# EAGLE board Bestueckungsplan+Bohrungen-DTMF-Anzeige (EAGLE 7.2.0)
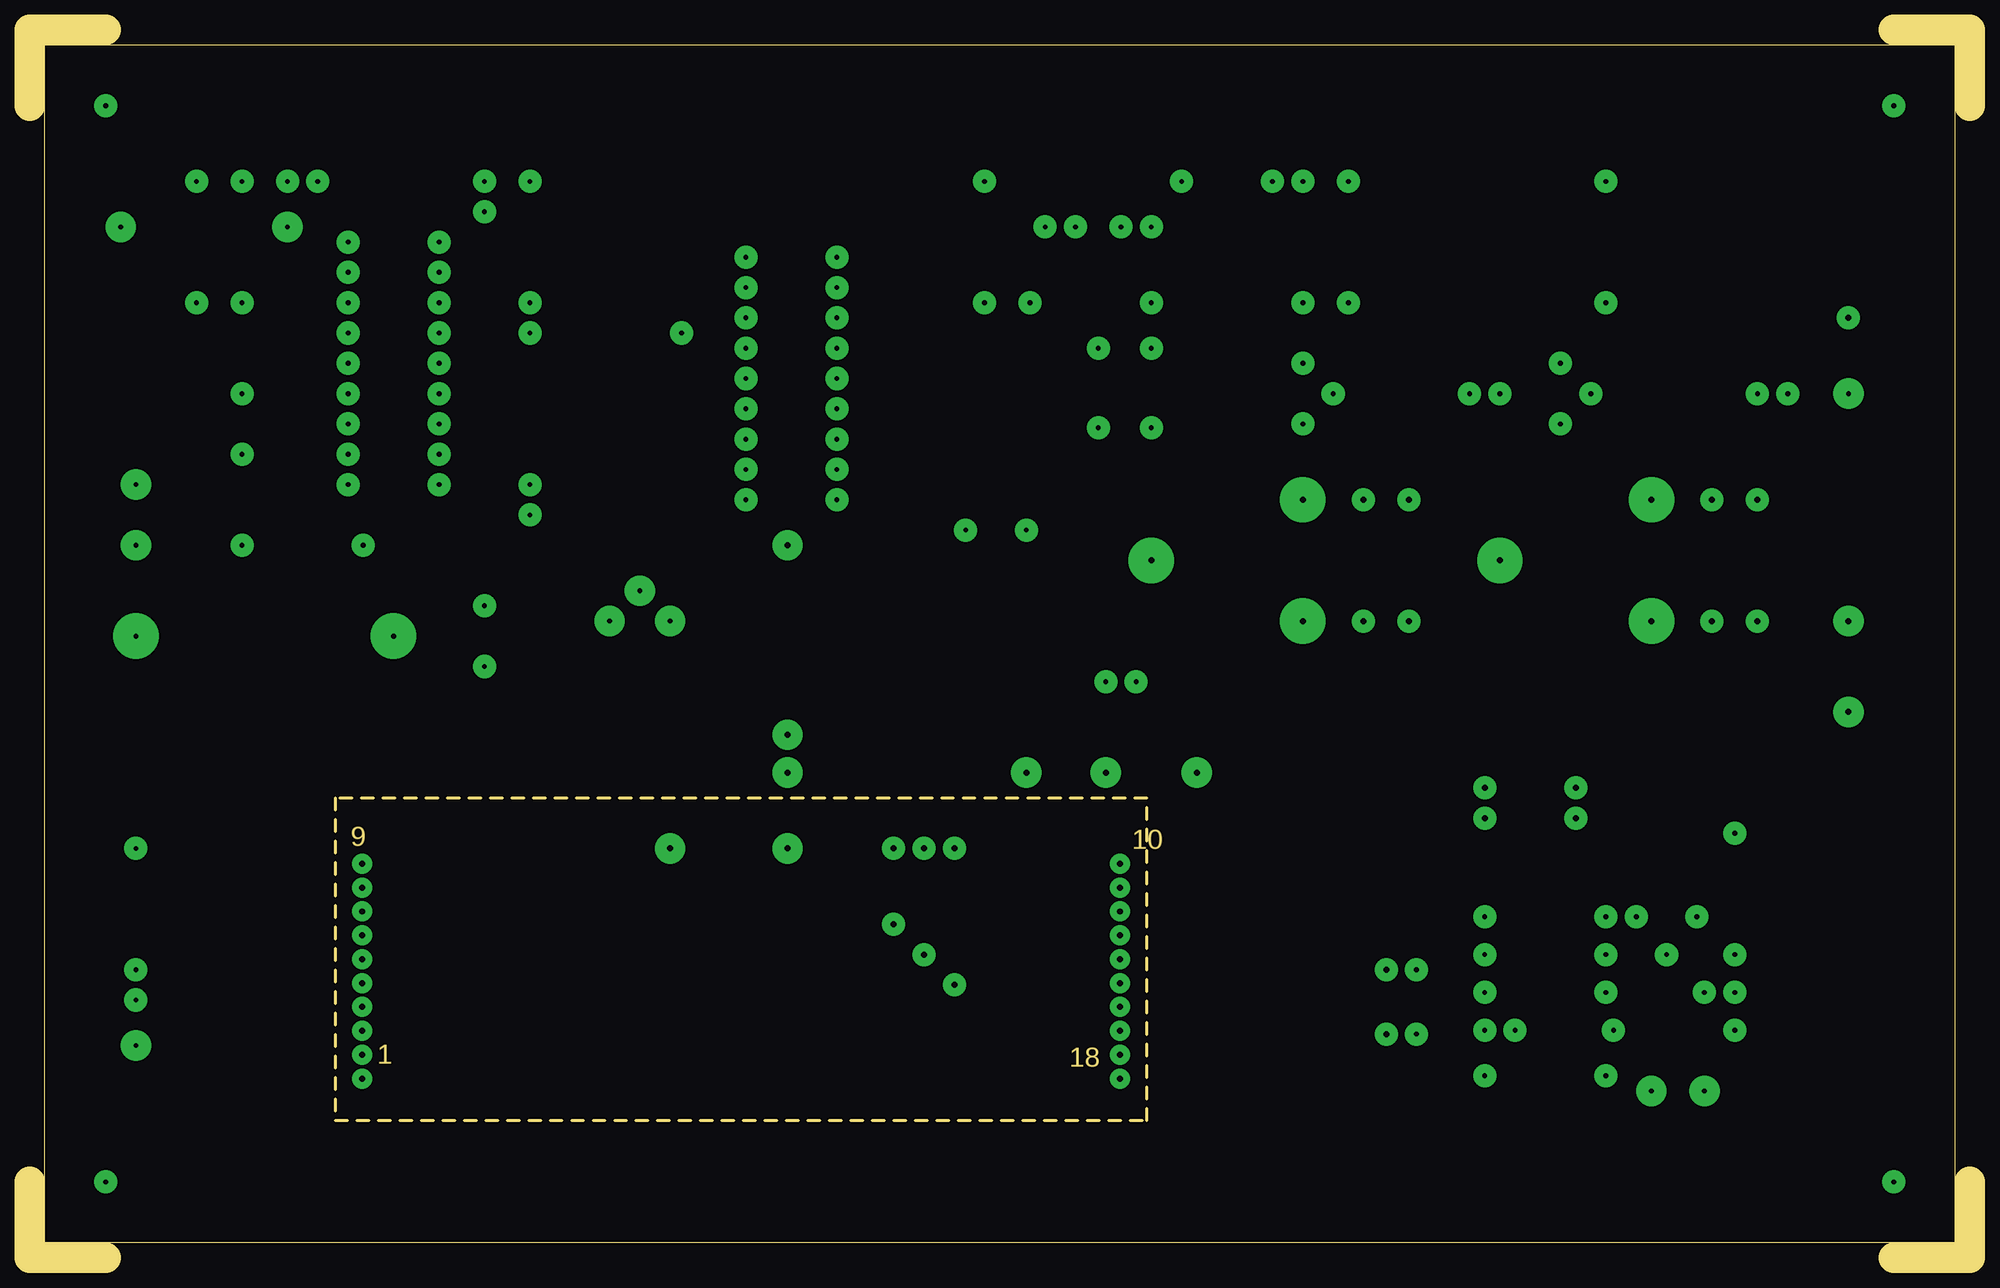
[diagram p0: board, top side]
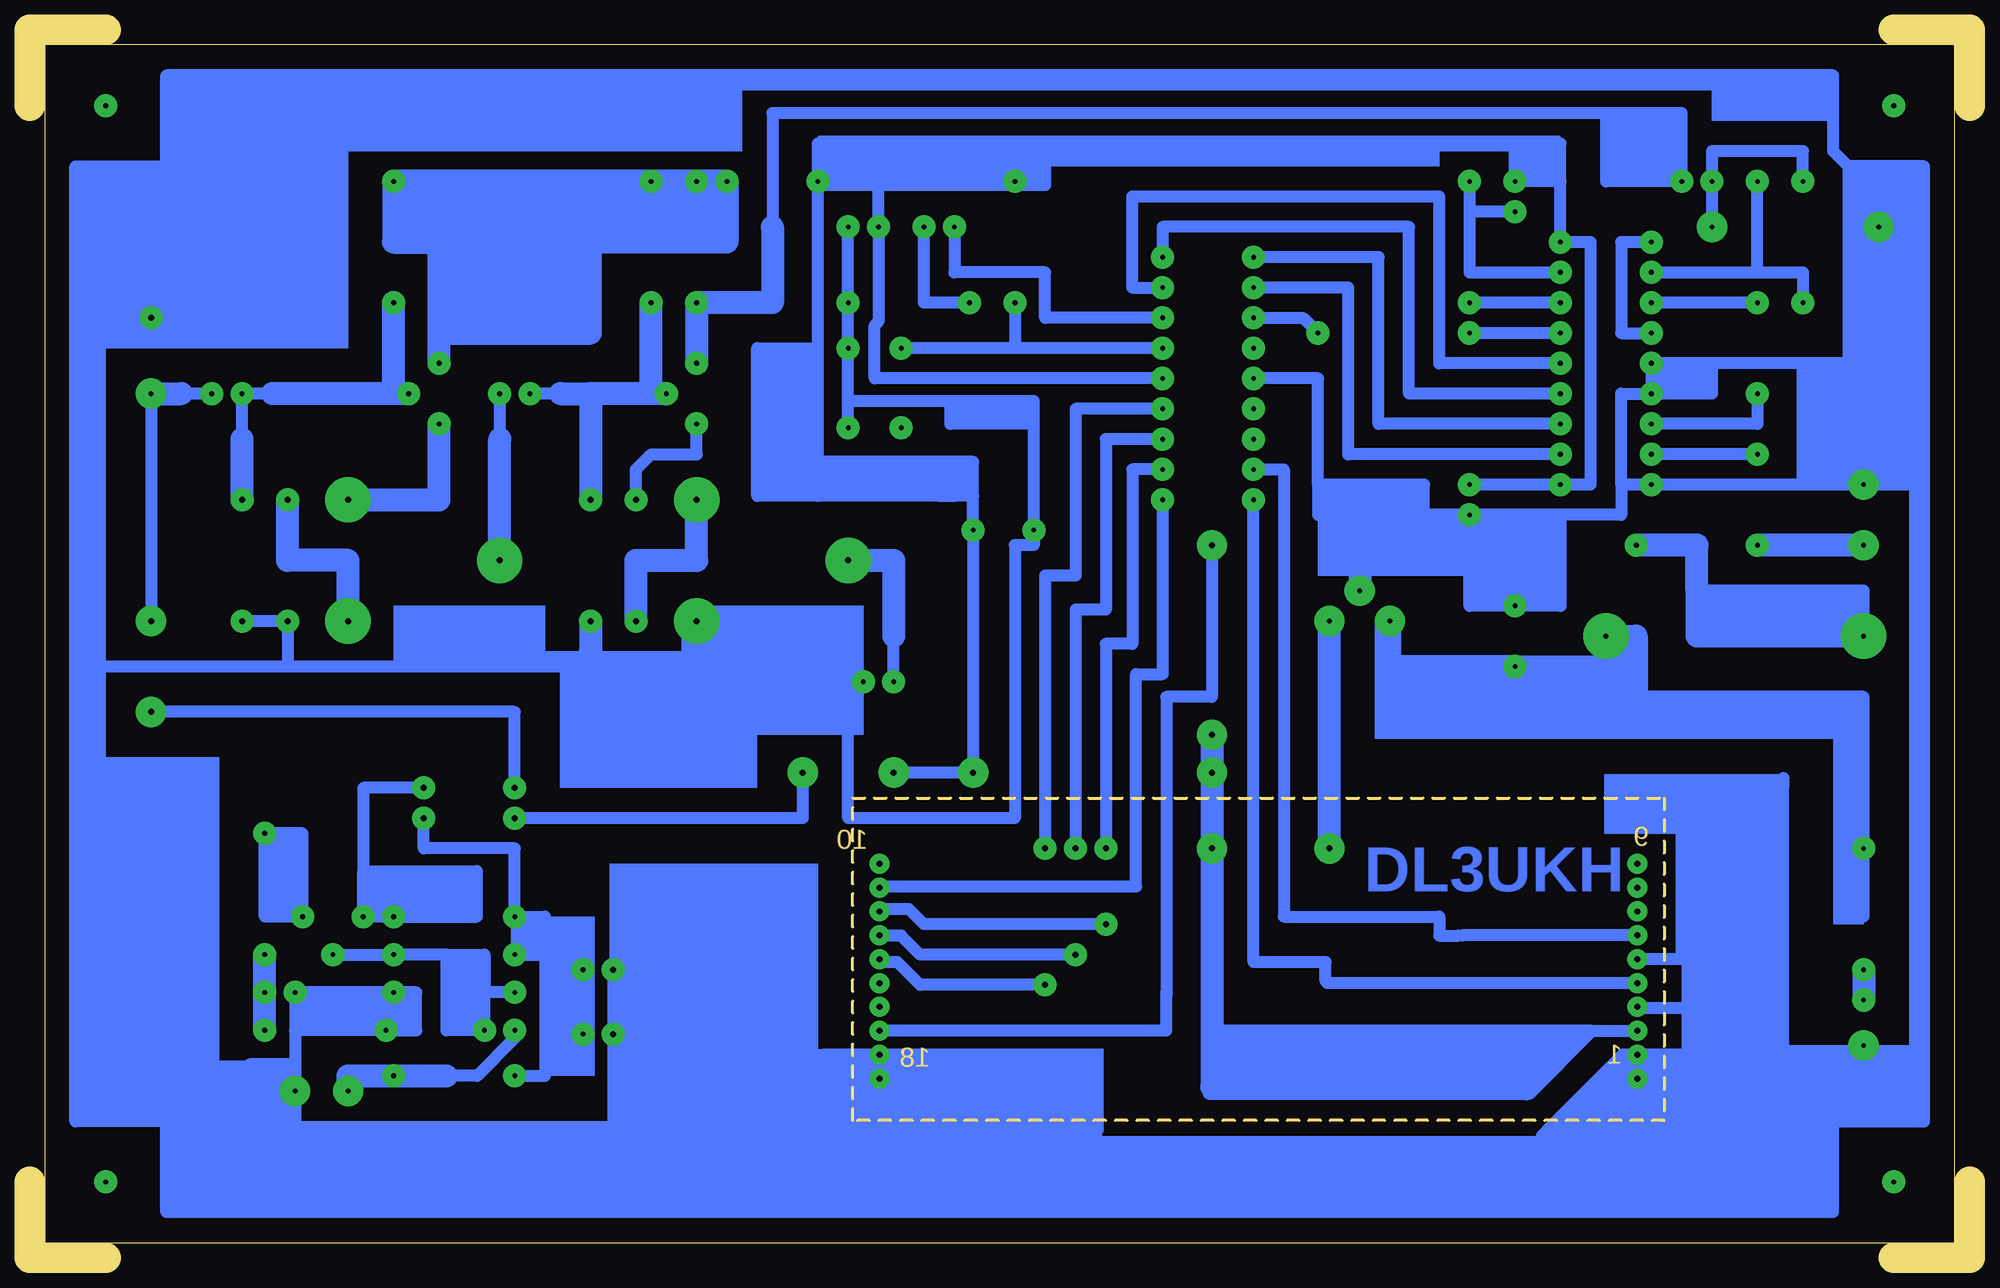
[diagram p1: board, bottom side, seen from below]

Size 162.56 x 102.87 mm. Coordinates in mm from the lower left corner, seen from the top.
Outline: 162.56,96.52 162.56,102.87 156.21,102.87
Outline: 162.56,6.35 162.56,0 156.21,0
Outline: 6.35,0 0,0 0,6.35
Outline: 0,96.52 0,102.87 6.35,102.87
Outline: 25.61,11.5 25.86,11.5
Outline: 25.61,11.5 93.6,11.5 93.6,38.51 25.61,38.51 25.61,11.5
Outline: 161.29,101.6 161.29,1.27 1.27,1.27 1.27,101.6 161.29,101.6
Copper layers (1*16): Top 0.035mm / dielectric 1.5mm / Bottom 0.035mm
Design rules "default": minimum track width 10mil, minimum drill 24mil, track to track 8mil, track to pad 8mil, pad to pad 8mil, via to via 8mil, smd to smd 8mil, copper to edge 40mil, drill to drill 8mil, minimum pad ring 10mil, minimum via ring 8mil, stop-mask expansion 4mil, vias tented up to drill 0mil, thermal gap 10mil

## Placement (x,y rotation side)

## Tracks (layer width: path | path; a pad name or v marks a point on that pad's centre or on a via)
S$1  (via drill 0.4 pad 1.93)
  other vias: 156.21,6.35
S$2  (via drill 0.4 pad 1.93)
  other vias: 156.21,96.52
S$3  (via drill 0.4 pad 1.93)
  other vias: 6.35,6.35
S$4  (via drill 0.4 pad 1.93)
  other vias: 6.35,96.52
S$5  (via drill 0.4 pad 1.93)
  other vias: 106.68,90.17
S$6  (via drill 0.4 pad 1.93)
  Bottom 1.016: v67.63,81.28 70.17,81.28 70.17,88.9 44.45,88.9 44.45,74.93 v34.29,74.93
S$7  (via drill 0.4 pad 1.93)
  Bottom 1.016: v80.01,90.17 81.28,93.03
S$8  (via drill 0.4 pad 1.93)
  Bottom 1.016: v67.63,76.2 80.01,76.2 | v80.01,80.01 80.01,76.2 | 80.01,76.2 v89.53,76.2 | v83.82,80.01 87.63,80.01 v87.63,86.36 | v67.63,78.74 77.47,78.74 77.47,82.55 85.09,82.55 v85.09,86.36
S$9  (via drill 0.4 pad 1.93)
  Bottom 1.016: 91.44,93.34 v91.44,86.36 91.44,78.42 91.76,78.1 91.76,73.66 v67.63,73.66
S$10  (via drill 0.4 pad 1.93, 0.4 pad 2.54)
  Bottom 1.016: v60.01,73.66 54.61,73.66 54.61,64.77 | 54.61,64.77 54.61,62.23 48.26,62.23 | 54.61,64.77 45.72,64.77 45.72,62.23 | 48.26,62.23 51.12,58.74 | 45.72,62.23 48.26,62.23 | v41.91,62.23 45.72,62.23 | v41.91,62.23 41.91,54.61 34.29,54.61 34.29,62.23 | 38.1,62.23 v41.91,62.23 | 38.1,62.23 38.1,58.42 | 34.29,62.23 38.1,62.23 | 34.29,62.23 29.21,62.23 29.21,64.77 | v26.67,72.39 29.21,72.39 29.21,64.77 | v26.67,72.39 21.59,72.39 21.59,74.93 | v26.67,72.39 v26.67,74.93 21.59,74.93 | 29.21,64.77 v26.67,64.77 13.97,64.77 | 13.97,64.77 13.97,74.93 | 10.16,74.93 13.97,74.93 | 10.16,74.93 7.62,74.93 | 13.97,74.93 21.59,74.93 | 10.16,91.44 11.43,92.71 11.43,99.06 151.13,99.06 151.13,91.44 158.75,91.44 158.75,50.8 | 10.16,91.44 10.16,74.93 | 10.16,64.77 13.97,64.77 | 10.16,64.77 10.16,74.93 | 10.16,64.77 v8.89,64.77 3.81,64.77 | 10.16,91.44 3.81,91.44 3.81,64.77 | 158.75,50.8 157.48,50.8 | 158.75,50.8 158.75,11.43 151.13,11.43 151.13,3.81 11.43,3.81 11.43,11.43 3.81,11.43 3.81,64.77
  Bottom 1.93: 51.12,58.74 v51.12,55.88 | 38.1,58.42 v38.1,54.61
S$11  (via drill 0.4 pad 1.93)
  other vias: 89.53,69.53
S$12  (via drill 0.4 pad 1.93)
  other vias: 60.01,68.58
S$13  (via drill 0.4 pad 1.93)
  other vias: 60.01,71.12
S$14  (via drill 0.4 pad 1.93)
  Bottom 1.016: 100.33,86.36 100.33,95.88 30.48,95.88 | 30.48,95.88 24.13,95.88 v24.13,90.17 30.48,90.17 30.48,95.88
  Bottom 1.93: v106.68,74.93 v106.68,80.01 100.33,80.01 100.33,86.36
S$15  (via drill 0.4 pad 1.93)
  Bottom 1.016: v93.98,86.36 v93.98,80.01 93.98,71.75 | v93.98,69.53 93.98,71.75 | 85.41,71.75 78.42,71.75 78.42,69.85 | 85.41,71.75 93.98,71.75 | 78.42,69.85 v78.42,60.96 78.42,59.69 80.01,59.69 80.01,36.83 93.98,36.83 93.98,44.45 | 78.42,69.85 85.41,69.85 85.41,71.75
S$16  (via drill 0.4 pad 2.54)
  other vias: 7.62,86.36
S$17  (via drill 0.4 pad 1.93)
  other vias: 93.98,76.2
S$18  (via drill 0.4 pad 1.93, 0.4 pad 3.81)
  Bottom 1.016: v8.89,52.07 8.89,55.88 22.86,55.88
  Bottom 1.93: v8.89,52.07 22.86,52.07 22.86,55.88 22.86,59.69 v27.94,59.69
S$19  (via drill 0.4 pad 1.93)
  Bottom 1.93: v8.89,24.13 v8.89,21.59
S$20  (via drill 0.5 pad 1.93)
  other vias: 152.4,78.74
S$21  (via drill 0.4 pad 1.93, 0.4 pad 2.54)
  Bottom 1.93: v8.89,59.69 v17.78,59.69
S$22  (via drill 0.4 pad 2.54)
  Bottom 1.93: 53.66,34.29 53.66,48.26 v53.66,53.34
S$23
  Bottom 1.016: 27.94,20.95 23.18,20.95
S$24  (via drill 0.4 pad 1.93, 0.4 pad 2.54)
  Bottom 1.016: v132.72,19.05 132.08,19.05 v132.08,22.22 | v132.08,22.22 v140.34,22.22 140.34,19.05 | v132.72,19.05 130.18,19.05 130.18,22.22 v132.08,22.22 | 140.34,19.05 v140.34,13.97 | v132.72,19.05 140.34,19.05 | v140.34,13.97 140.34,11.43 | 140.34,11.43 140.34,10.16 | 140.34,11.43 144.15,11.43 | 144.15,11.43 144.15,10.16 140.65,10.16 | v140.34,13.97 140.34,16.19 144.15,16.19 144.15,11.43
S$25  (via drill 0.4 pad 1.93)
  other vias: 60.01,66.04
S$26  (via drill 0.5 pad 1.93, 0.5 pad 2.54)
  Bottom 1.016: v121.92,39.37 121.92,45.72 v152.4,45.72
S$27  (via drill 0.5 pad 1.68)
  other vias: 27.86,21
S$28  (via drill 0.5 pad 1.68)
  Bottom 1.016: v27.86,31 27.81,31 27.81,31.06
S$29  (via drill 0.4 pad 1.93)
  Bottom 1.016: 38.1,93.34 v38.1,90.17 34.29,90.17 | 34.29,90.17 34.29,93.34 | 34.29,90.17 v34.29,85.09 31.75,85.09 31.75,64.77 v34.29,64.77 v41.91,64.77
S$30  (via drill 0.5 pad 1.68)
  Bottom 1.016: 91.21,31.07 91.21,31 v91.35,31
S$31  (via drill 0.5 pad 1.68)
  Bottom 1.016: 91.17,28.85 91.17,29 v91.35,29
S$32  (via drill 0.4 pad 1.93, 0.4 pad 2.54, 0.5 pad 2.54)
  Bottom 1.016: v147.32,72.39 149.86,72.39 | v152.4,72.39 v152.4,53.34
  Bottom 1.93: v152.4,72.39 149.86,72.39
S$33  (via drill 0.4 pad 1.93, 0.5 pad 1.93)
  Bottom 1.016: v67.63,66.04 70.17,66.04 70.17,51.44 72.39,51.44 v72.39,34.29
S$34  (via drill 0.4 pad 1.93, 0.5 pad 1.93)
  Bottom 1.016: v67.63,68.58 72.39,68.58 72.39,54.29 74.93,54.29 v74.93,34.29
S$35  (via drill 0.4 pad 1.93, 0.5 pad 1.93)
  Bottom 1.016: v67.63,71.12 74.93,71.12 74.93,57.15 77.47,57.15 v77.47,34.29
S$36  (via drill 0.4 pad 2.54)
  other vias: 8.89,17.78
S$37  (via drill 0.5 pad 1.68)
  Bottom 1.016: 91.45,26.94 91.45,27 v91.35,27
S$38  (via drill 0.5 pad 1.68)
  Bottom 1.016: 91.41,25.04 91.41,25 v91.35,25
S$39  (via drill 0.4 pad 1.93, 0.5 pad 3.81)
  Bottom 1.016: v123.19,72.39 123.19,68.58
  Bottom 1.93: v123.19,58.42 123.19,68.58
S$40  (via drill 0.5 pad 1.68)
  Bottom 1.016: 91.39,33.03 91.39,32.93 91.35,32.93 v91.35,33.01
S$41
  Bottom 1.016: 60.01,66.04 57.47,66.04 57.47,28.57 44.45,28.57 44.45,26.99 42.86,26.99
S$42  (via drill 0.4 pad 1.93, 0.5 pad 1.93)
  Bottom 1.016: v111.76,63.5 111.76,66.04 110.49,67.31 106.68,67.31 v106.68,69.85
S$43  (via drill 0.5 pad 1.93, 0.5 pad 3.81)
  Bottom 1.93: v111.76,53.34 111.76,58.42 106.68,58.42 v106.68,63.5
S$44  (via drill 0.4 pad 1.93, 0.5 pad 1.93, 0.5 pad 3.81)
  Bottom 1.016: v92.71,48.26 95.25,48.26 96.52,49.53 106.68,49.53 | 106.68,50.8 106.68,49.53 | v144.78,53.34 v140.97,53.34 140.97,49.53 | 115.57,50.8 115.57,49.53 | 115.57,49.53 140.97,49.53 | 140.97,49.53 156.21,49.53 | 106.68,49.53 115.57,49.53
  Bottom 1.93: v106.68,53.34 106.68,50.8 | v115.57,53.34 115.57,50.8
S$45  (via drill 0.4 pad 1.93, 0.5 pad 3.81)
  Bottom 1.016: v90.17,48.26 90.17,52.07
  Bottom 1.93: v93.98,58.42 90.17,58.42 90.17,52.07
S$46  (via drill 0.4 pad 1.93, 0.5 pad 1.93)
  Bottom 1.016: 118.11,72.39 v120.65,72.39
  Bottom 1.93: v110.49,80.01 110.49,72.39 v109.22,72.39 115.57,72.39 | 118.11,72.39 115.57,72.39 | 115.57,72.39 v115.57,63.5
S$47  (via drill 0.5 pad 1.68)
  Bottom 1.016: 27.77,29.16 27.77,29 v27.86,29
S$48  (via drill 0.5 pad 1.68)
  Bottom 1.016: 53.27,16.15 53.27,16.25 63.79,13.75 36.86,13.75 31.61,19 v27.86,19
S$49  (via drill 0.5 pad 1.68)
  Bottom 1.016: 91.58,19.09 91.58,19 v91.35,19
S$50  (via drill 0.4 pad 1.93)
  Bottom 1.016: v26.67,82.55 17.78,82.55 | 17.78,82.55 v17.78,90.17 | 17.78,82.55 13.97,82.55 v13.97,80.01
S$51  (via drill 0.4 pad 1.93)
  Bottom 1.016: v26.67,85.09 29.21,85.09 29.21,77.47 v26.67,77.47
S$52  (via drill 0.4 pad 1.93, 0.5 pad 3.81)
  Bottom 1.93: v135.89,63.5 128.27,63.5 v128.27,69.85
S$53  (via drill 0.5 pad 1.68)
  other vias: 27.86,15
S$54  (via drill 0.5 pad 1.68)
  Bottom 1.016: v91.35,15 95.22,15
S$55  (via drill 0.5 pad 1.68)
  Bottom 1.016: v27.86,33.01 28.17,33.01 28.17,32.97
S$56  (via drill 0.5 pad 1.93, 0.5 pad 3.81)
  Bottom 1.93: v135.89,53.34 135.89,58.42 140.97,58.42 v140.97,63.5
S$59
  Bottom 1.016: 15.56,10.48 15.56,9.84 35.88,9.84 | 35.88,9.84 35.88,10.16 33.66,12.38 | 35.88,9.84 35.88,4.13
S$60  (via drill 0.5 pad 2.54)
  other vias: 53.66,34.29
S$61  (via drill 0.5 pad 2.54)
  Bottom 1.93: v63.5,43.82 v63.5,40.64 v63.5,34.29 63.5,14.29
S$62
  Bottom 1.016: 37.15,13.65 37.15,13.97
S$63  (via drill 0.5 pad 1.68)
  other vias: 27.86,21
S$64  (via drill 0.5 pad 1.68)
  other vias: 27.86,25
S$65  (via drill 0.5 pad 1.68)
  Bottom 1.016: v91.35,17 95.22,17
S$66  (via drill 0.5 pad 1.68)
  other vias: 91.35,21
S$67  (via drill 0.5 pad 1.68)
  other vias: 91.35,23
S$68  (via drill 0.4 pad 1.93, 0.5 pad 1.93)
  Bottom 1.016: 142.24,72.39 v144.78,72.39 144.78,68.58
  Bottom 1.93: 132.08,72.39 v132.08,80.01 | 132.08,72.39 142.24,72.39 | v130.81,72.39 132.08,72.39 | v144.78,63.5 144.78,68.58
S$69  (via drill 0.5 pad 1.68)
  Bottom 1.016: v27.86,31 27.81,31 27.81,31.06
S$70  (via drill 0.5 pad 1.68)
  Bottom 1.016: 91.53,31.07 91.21,31 v91.35,31
S$71  (via drill 0.5 pad 1.68)
  Bottom 1.016: 91.49,28.85 91.49,29 v91.35,29
S$72  (via drill 0.5 pad 1.68)
  Bottom 1.016: 91.45,26.94 91.45,27 v91.35,27
S$73  (via drill 0.5 pad 1.68)
  Bottom 1.016: 91.41,25.04 91.41,25 v91.35,25
S$74  (via drill 0.5 pad 1.68)
  Bottom 1.016: 91.39,33.03 91.39,32.93 91.35,32.93 v91.35,33.01
S$75  (via drill 0.5 pad 1.68)
  Bottom 1.016: 27.77,29.16 27.77,29 v27.86,29
S$76  (via drill 0.5 pad 1.68)
  Bottom 1.016: 53.27,16.15 53.27,16.25 58.71,13.75 53.11,13.75 | 53.11,13.75 36.86,13.75 31.61,19 | 31.61,19 v27.86,19 | 31.61,19 53.11,19 53.11,13.75
S$77  (via drill 0.5 pad 1.68)
  Bottom 1.016: 91.26,19.09 91.26,19 v91.35,19
S$78  (via drill 0.5 pad 1.68)
  Bottom 1.016: v91.35,15 95.22,15
S$79  (via drill 0.5 pad 1.68)
  Bottom 1.016: v27.86,33.01 v27.85,33.01 27.85,32.97
S$82  (via drill 0.5 pad 1.68)
  other vias: 27.86,23
S$83  (via drill 0.5 pad 1.68)
  other vias: 27.86,23 27.86,23
S$84  (via drill 0.5 pad 1.68)
  other vias: 27.86,27
S$85  (via drill 0.5 pad 2.54)
  Bottom 1.016: v63.5,59.69 63.5,46.99 67.31,46.99 67.31,22.22 67.31,21.91 67.31,19.05 91.44,19.05
S$86  (via drill 0.4 pad 1.93)
  Bottom 1.016: 91.44,31.11 69.85,31.11 69.85,48.9 67.63,48.9 v67.63,63.5
S$87  (via drill 0.5 pad 1.93)
  Bottom 1.016: v72.39,27.94 87.63,27.94 88.9,29.21 91.44,29.21
S$88  (via drill 0.5 pad 1.93)
  Bottom 1.016: v113.66,24.13 113.66,4.13
S$89  (via drill 0.4 pad 1.68)
  Bottom 1.016: v27.86,25 27.82,25 27.82,25.34 27.73,25.03
  other vias: 27.86,21
S$90  (via drill 0.4 pad 1.68)
  Bottom 1.016: v91.35,17 94.58,17
S$91  (via drill 0.4 pad 1.68)
  other vias: 91.35,21
S$92  (via drill 0.4 pad 1.68)
  other vias: 91.35,23
S$93  (via drill 0.4 pad 1.68)
  Bottom 1.016: v27.86,31 27.81,31 27.81,31.06
S$94  (via drill 0.4 pad 1.68)
  Bottom 1.016: 91.53,31.07 91.21,31 v91.35,31
S$95  (via drill 0.4 pad 1.68)
  Bottom 1.016: 91.17,28.85 91.17,29 v91.35,29
S$96  (via drill 0.4 pad 1.68)
  Bottom 1.016: 91.45,26.94 91.45,27 v91.35,27
S$97  (via drill 0.4 pad 1.68)
  Bottom 1.016: 91.41,25.04 91.09,25 v91.35,25
S$98  (via drill 0.4 pad 1.68)
  Bottom 1.016: 91.39,33.03 91.39,32.93 91.35,32.93 v91.35,33.01
S$99  (via drill 0.4 pad 1.68)
  Bottom 1.016: 27.77,29.16 27.77,29 v27.86,29
S$100  (via drill 0.4 pad 1.68)
  Bottom 1.016: 53.27,16.15 52.95,16.25 59.98,13.75 53.11,13.75 | 53.11,13.75 36.86,13.75 31.61,19 | 31.61,19 v27.86,19 | 31.61,19 53.11,19 53.11,13.75
S$101  (via drill 0.4 pad 1.93)
  Bottom 1.93: 128.27,90.17 v110.49,90.17 v104.14,90.17 104.14,85.09 127,85.09 | 128.27,90.17 v132.08,90.17 132.08,85.09 127,85.09 | v128.27,74.93 128.27,77.47 | 128.27,77.47 128.27,85.09 | 128.27,85.09 128.27,90.17 | 127,85.09 128.27,85.09 | 128.27,77.47 115.57,77.47 115.57,86.36
S$102  (via drill 0.4 pad 1.93)
  Bottom 1.016: v34.29,80.01 v41.91,80.01
S$103  (via drill 0.4 pad 1.93)
  Bottom 1.016: v34.29,77.47 v41.91,77.47
S$104  (via drill 0.4 pad 1.68)
  Bottom 1.016: 91.26,19.09 91.26,19 v91.35,19
S$105  (via drill 0.4 pad 1.93)
  Bottom 1.016: v34.29,72.39 46.99,72.39 46.99,86.36 67.63,86.36 v67.63,83.82
S$106  (via drill 0.4 pad 1.93)
  Bottom 1.016: v34.29,69.85 49.53,69.85 49.53,83.82 v60.01,83.82
S$107  (via drill 0.4 pad 1.93)
  Bottom 1.016: v34.29,67.31 52.07,67.31 52.07,81.28 v60.01,81.28
S$108  (via drill 0.4 pad 1.93)
  Bottom 1.016: v60.01,78.74 55.88,78.74 v54.61,77.47
S$109  (via drill 0.4 pad 1.68)
  Bottom 1.016: v91.35,15 95.22,15
S$110  (via drill 0.4 pad 1.93)
  other vias: 60.01,76.2
S$111  (via drill 0.4 pad 1.68)
  Bottom 1.016: v27.86,33.01 v27.85,33.01 27.85,32.97
S$113  (via drill 0.4 pad 1.68)
  Bottom 1.016: v27.86,23 53.86,23 53.86,23.12
S$114  (via drill 0.4 pad 1.68)
  Bottom 1.016: v27.86,23 36.11,23
S$115  (via drill 0.4 pad 1.93)
  Bottom 1.016: v41.91,90.17 41.91,87.63 | 41.91,87.63 41.91,82.55 v34.29,82.55 | v38.1,87.63 41.91,87.63
S$116  (via drill 0.4 pad 1.68)
  Bottom 1.016: v27.86,27 42.54,27
S$117  (via drill 0.4 pad 1.93)
  Bottom 1.016: 116.2,26.99 v116.2,24.13 v116.2,18.73 | 116.2,15.88 v116.2,18.73 | v116.2,18.73 116.2,25.4
S$118  (via drill 0.4 pad 1.93)
  Bottom 1.016: v17.78,67.31 v26.67,67.31
S$119  (via drill 0.4 pad 1.93)
  Bottom 1.016: v17.78,72.39 17.78,69.85 v26.67,69.85
S$120  (via drill 0.4 pad 1.93)
  Bottom 1.016: v17.78,80.01 v26.67,80.01
S$121  (via drill 0.4 pad 1.68)
  Bottom 1.016: 34.11,11 30.11,15 v27.86,15 v27.86,17 29.11,17 35.36,10.75
S$123  (via drill 0.4 pad 1.93, 0.4 pad 2.54)
  Bottom 1.016: v13.97,90.17 13.97,92.71 21.59,92.71 v21.59,90.17 v21.59,86.36
S$124  (via drill 0.5 pad 1.68)
  Bottom 1.016: 34.11,11 30.11,15 v27.86,15 v27.86,17 29.11,17 35.36,10.75
S$125  (via drill 0.5 pad 1.93)
  Bottom 1.016: v74.93,25.4 87.95,25.4 89.53,26.99 91.44,26.99
S$126  (via drill 0.5 pad 1.93)
  Bottom 1.016: v77.47,22.86 87.95,22.86 89.85,24.77 91.44,24.77
S$127  (via drill 0.4 pad 1.93)
  Bottom 1.016: 96.52,93.34 v96.52,90.17 96.52,89.85 | 96.52,76.2 96.52,89.85 | 96.52,63.82 96.52,66.67 | 96.52,66.67 96.52,76.2 | 96.52,76.2 101.6,76.2 101.6,63.82 86.36,63.82 | 86.36,63.82 85.09,63.82 | 77.47,91.44 77.47,89.85 96.52,89.85 | 86.36,63.82 86.36,66.67 | 86.36,66.67 96.52,66.67 | 85.09,63.82 85.09,66.67 | 85.09,66.67 86.36,66.67 | 83.5,63.82 v83.5,60.96 83.5,40.64 | 83.5,63.82 85.09,63.82 | 83.5,63.82 83.5,66.67 85.09,66.67
S$128  (via drill 0.5 pad 2.54)
  Bottom 1.016: v83.5,40.64 v90.17,40.64
S$129  (via drill 0.4 pad 1.68)
  Bottom 1.016: 27.93,21 v27.86,21 | 15.86,25 16.61,25 | 16.61,25 27.82,25 | v27.86,25 27.82,25 | 27.82,25 27.82,25.03 27.73,25.03 | 34.11,11 30.11,15 v27.86,15 | 35.36,10.75 29.11,17 v27.86,17 | v27.86,15 22.86,15 | v27.86,17 v27.86,15 | 23.61,17 v27.86,17 | 23.61,17 16.61,17 | 16.61,17 16.11,17 | 23.61,10.39 23.61,17 | 16.61,25 16.61,17
S$130  (via drill 0.4 pad 1.93, 0.4 pad 2.54, 0.4 pad 3.81)
  Bottom 1.016: v38.1,49.53 38.1,45.72 11.43,45.72 11.43,46.99 | 11.43,46.99 29.21,46.99 | 11.43,46.99 8.89,46.99 v8.89,34.29 | v8.89,34.29 10.16,34.29 | 8.89,30.48 v8.89,34.29 | 8.89,30.48 10.79,30.48 | 8.89,28.57 8.89,30.48
  Bottom 1.93: 27.94,46.99 27.94,52.07 v30.48,52.07 30.48,49.53 v38.1,49.53 48.58,49.53 | 48.58,49.53 v48.58,53.34 | 48.58,49.53 48.58,46.99
S$131  (via drill 0.4 pad 1.68)
  Bottom 1.016: v91.35,17 95.22,17
S$132  (via drill 0.4 pad 1.68)
  other vias: 91.35,21
S$133  (via drill 0.4 pad 1.68)
  other vias: 91.35,23
S$134  (via drill 0.4 pad 1.68)
  Bottom 1.016: v27.86,31 27.81,31 27.81,31.06
S$135  (via drill 0.4 pad 1.68)
  Bottom 1.016: 91.21,31.07 91.21,31 v91.35,31
S$136  (via drill 0.4 pad 1.68)
  Bottom 1.016: 91.17,28.85 91.49,29 v91.35,29
S$137  (via drill 0.4 pad 1.68)
  Bottom 1.016: 91.45,26.94 91.45,27 v91.35,27
S$138  (via drill 0.4 pad 1.68)
  Bottom 1.016: 91.41,25.04 91.41,25 v91.35,25
S$139  (via drill 0.4 pad 1.68)
  Bottom 1.016: 91.39,33.03 91.39,33.24 91.35,33.24 v91.35,33.01
S$140  (via drill 0.4 pad 1.68)
  Bottom 1.016: 27.77,29.16 27.77,29 v27.86,29
S$141  (via drill 0.4 pad 1.68)
  Bottom 1.016: 53.27,16.15 53.91,16.25 59.03,13.75 53.11,13.75 | 53.11,13.75 36.86,13.75 31.61,19 | 31.61,19 v27.86,19 | 31.61,19 63.58,19 53.11,13.75
S$142  (via drill 0.4 pad 1.68)
  Bottom 1.016: 91.26,19.09 91.26,19 v91.35,19
S$143  (via drill 0.4 pad 1.68)
  Bottom 1.016: v91.35,15 94.58,15
S$144  (via drill 0.4 pad 1.68)
  Bottom 1.016: v27.86,33.01 v27.85,33.01 27.85,32.97
S$146  (via drill 0.4 pad 1.68)
  Bottom 1.016: v27.86,23 53.54,23 53.86,23.12
S$147  (via drill 0.4 pad 1.68)
  Bottom 1.016: v27.86,23 36.11,23
S$148  (via drill 0.4 pad 1.68)
  other vias: 27.86,27
S$149  (via drill 0.4 pad 1.93)
  Bottom 1.016: v139.7,28.57 139.7,35.56 v142.88,35.56 142.88,28.57 v139.7,28.57
S$151  (via drill 0.4 pad 1.93)
  Bottom 1.016: v142.88,25.4 v142.88,22.22 v142.88,19.05
  Bottom 1.93: v142.88,19.05 v142.88,25.4
S$152
  Bottom 1.016: 15.61,10.46 15.61,39.55
S$153
  Bottom 1.016: 15.61,10.46 15.61,39.87
S$154
  Bottom 1.016: 15.61,10.78 15.61,40.19
S$155  (via drill 0.4 pad 1.93)
  Bottom 1.016: 53.98,23.18 53.98,24.77 60.01,24.77 v60.01,63.5
S$156  (via drill 0.4 pad 1.93)
  Bottom 1.016: v121.92,22.22 124.46,22.22 | 124.46,22.22 127.63,22.22 | 127.63,22.22 127.63,25.4 | v137.16,25.4 v132.08,25.4 127.63,25.4 | 127.63,22.22 127.63,19.05 v124.46,19.05 124.46,22.22 | 127.63,25.4 124.46,25.4 124.46,22.22
S$157  (via drill 0.4 pad 1.93, 0.4 pad 2.54)
  Bottom 1.016: v121.92,19.05 121.92,18.41 125.09,15.24 127.63,15.24 v132.08,15.24 135.89,15.24
  Bottom 1.93: v135.89,13.97 135.89,15.24 127.63,15.24
S$158  (via drill 0.5 pad 1.93)
  other vias: 113.66,18.73
S$160  (via drill 0.4 pad 1.93, 0.5 pad 1.93)
  Bottom 1.016: 119.38,25.4 119.38,28.57 v121.92,28.57 121.92,34.29 129.54,34.29 v129.54,36.83 | 119.38,25.4 119.38,15.24 v121.92,15.24 | v121.92,25.4 119.38,25.4
S$161  (via drill 0.4 pad 1.93, 0.5 pad 1.93)
  Bottom 1.016: 134.62,32.38 134.62,31.75 v134.62,28.57 v132.08,28.57 125.09,28.57 125.09,32.38 134.62,32.38 | v129.54,39.37 134.62,39.37 134.62,32.38
S$163  (via drill 0.5 pad 1.93, 0.5 pad 2.54)
  Bottom 1.016: v97.79,40.64 97.79,36.83 v121.92,36.83
(copper drawn outside any net)
  shapes: Bottom area x97

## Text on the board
Bottom: DL3UKH
Pads: AUF BESTÜCKUNGS-SEITE GESEHEN
Dimension: 9 | 10 | 1 | 18
tOrigins: 7805 | BC547C | 1N4002 | LED rot/grün | IC's | 1 | Leiterplatte: | Die Aussparung | 1,5mm dick | Links oben ist | muß mit dem | immer PIN 1 | Bauelement | Cevausit | und dem Bestück- | ungsplan | Katode | Anode | überein stimmen. | Kat | Eing. | Ausg. | K | wie | K | E | Masse | Katode | Alles mit 0,8mm vorbohren ! | B | Anode | Aufbohren: | immer an + Pol | Diode 1N4002 1,0mm | Sicherungshalter 1,5mm | Anschluß-Drähte 1,0mm | 4Stck. Befestigungsbohr... 3,2mm | Einstellregler 1,2mm | 100n | Brücke | µA7805 1,0mm | 300mV | NF-Messpunkt | LED rt | 100n | K | 1 | 1 | 47n | 100K | 100K | 330K | 10K | 33K | 2,2M | 1,0M | 2,2K | Die 8 Brücken | Brücke | K | nicht vergessen ! | Masse | K | 4,7µ | 4,7µ | Taster | BC547 | Masse | + | + | MT8870 | BC547 | Masse | Quarz | E | PIC16F88 | E | 1N4002 | 47n | + | + 12Volt | Masse | 100K | NF-Eingang | 470µ/25V | 10K | Kat | 820 | 3,3M | 390K | 6,2K | Sicherungs- | Eing. | Ausg. | 4,7µ | Halter | + | 470µ/25V | + | 12ohm | 7805 | Brücke | Brücke | DIL | Brücke | Steht für den | Pluspol eines | 4,7 | BC547c | Brücke | Elkos oder | C | E | Brücken | 470 | Tantal-Kond. | 6,2K | 20K | B | + ist immer | 100µ/16V | 4,7µ | + | 6,2K | + | langer Draht | 100µ/16V | + | 100 | 4,7µ | wenn bei Tantal | + | 1 | beide Drähte | LED gn | K | 7,5K | 2 | gleich sind ist | Mikrophon | es egal | ACHTUNG zum LCD-Display : | Es sind bei der LCD-Anzeige 9 Stifte aber die Buchsenleiste hat 10 Buchsen ! | Und auch richtig herum reinstecken. | Die Zahlen auf dem Bestückungsplan und auf dem LCD-Display müssen überein stimmen !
